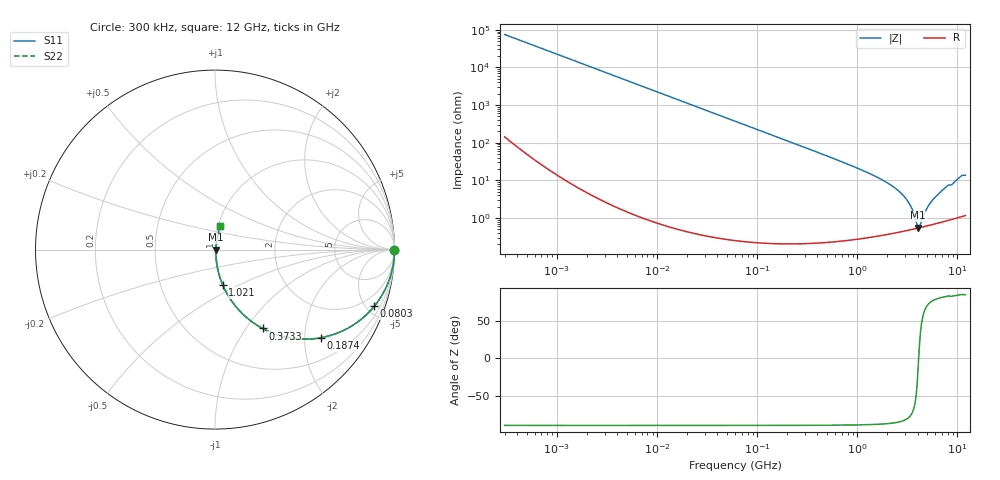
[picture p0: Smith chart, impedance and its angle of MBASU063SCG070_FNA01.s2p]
! MBASU063SCG070_FNA01  S-PARAMETER MODEL  ( Standard Model )
! Model Generated by TAIYO YUDEN Corporation (http://www.ty-top.com)
! Version 1.0
! TAIYO YUDEN Control No. 230609
! Copyright(c) 2023 TAIYO YUDEN CO.,LTD. All Rights Reserved.
! Product Description (link to TY-COMPAS)
! https://ds.yuden.co.jp/TYCOMPAS/or/detail?pn=MBASU063SCG070CFNA01&u=M
! Products Name : Multilayer Ceramic Capacitors
! Characteristics :
!  Capacitance : 7 [pF] , Rated Voltage : 50 [V] , TCC : CG / C0G
!  Case Size : 0.6 x 0.3 / 0.024 x 0.012 [mm/inch] , Thickness : 0.3 / 0.012 [mm/inch]
!  (Conditions: Temperature = 25 [degC] , DC Bias Voltage = 0 [V])
! External Node Assignments :
!  1  o---| |---o  2
! GND o---------o GND
! Frequency Range : 0.3MHz  -  12000MHz  [ 401 STEP ]
# MHZ S RI R 50
! Freq[MHz].  S11 Real  S11 Imag  S21 Real  S21 Imag  S12 Real  S12 Imag  S22 Real  S22 Imag
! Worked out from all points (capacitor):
!   401 points, 300 kHz to 12 GHz, reference 50 ohm
!   read as one part in series: C = 7.06 pF near 316.3 kHz
!   lowest |Z| = 552 mohm at 4.05 GHz (marker M1)
!   series resonance near 4.093 GHz, so ESL is about 210 pH
!   S11 on the Smith chart (normalised r, x): 300 kHz: open; 80.3 MHz: 1.00, -5.61; 187.4 MHz: 1.00, -2.40; 373.3 MHz: 1.00, -1.20; 1.021 GHz: 1.01, -0.41; 12 GHz: 1.02, +0.27
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0.3  1 -0.00133  4.32e-06 0.00133  4.32e-06 0.00133  1 -0.00133
1.769972  0.9999 -0.00785  6.51e-05 0.00785  6.51e-05 0.00785  0.9999 -0.00785
10.44266  0.9978 -0.0462  0.00216 0.0462  0.00216 0.0462  0.9978 -0.0462
27.10171  0.9857 -0.1185  0.0143 0.1185  0.0143 0.1185  0.9857 -0.1185
60  0.9337 -0.2485  0.0663 0.2485  0.0663 0.2485  0.9337 -0.2485
80.29859  0.8871 -0.3161  0.1129 0.3161  0.1129 0.3161  0.8871 -0.3161
187.4445  0.59 -0.491  0.41 0.491  0.41 0.491  0.59 -0.491
353.9943  0.2861 -0.4502  0.7139 0.4502  0.7139 0.4502  0.2861 -0.4502
373.2558  0.2647 -0.4394  0.7353 0.4394  0.7353 0.4394  0.2647 -0.4394
601.3112  0.1201 -0.3219  0.8799 0.3219  0.8799 0.3219  0.1201 -0.3219
1021.415  0.0435 -0.1974  0.9565 0.1974  0.9565 0.1974  0.0435 -0.1974
2088.533  0.01 -0.0787  0.99 0.0787  0.99 0.0787  0.01 -0.0787
2650.866  0.00663 -0.0489  0.9934 0.0489  0.9934 0.0489  0.00663 -0.0489
3107.553  0.00555 -0.0304  0.9944 0.0304  0.9944 0.0304  0.00555 -0.0304
3454.93  0.00526 -0.0186  0.9947 0.0186  0.9947 0.0186  0.00526 -0.0186
3944.255  0.00533 -0.00407  0.9947 0.00407  0.9947 0.00407  0.00533 -0.00407
4050.141  0.0054 -0.000974  0.9946 0.000974  0.9946 0.000974  0.0054 -0.000974
4270.516  0.0056 0.00385  0.9944 -0.00385  0.9944 -0.00385  0.0056 0.00385
5140.631  0.0067 0.0204  0.9933 -0.0204  0.9933 -0.0204  0.0067 0.0204
6188.031  0.00857 0.038  0.9914 -0.038  0.9914 -0.038  0.00857 0.038
10511.28  0.0242 0.1162  0.9758 -0.1162  0.9758 -0.1162  0.0242 0.1162
12000  0.0292 0.1309  0.9708 -0.1309  0.9708 -0.1309  0.0292 0.1309
